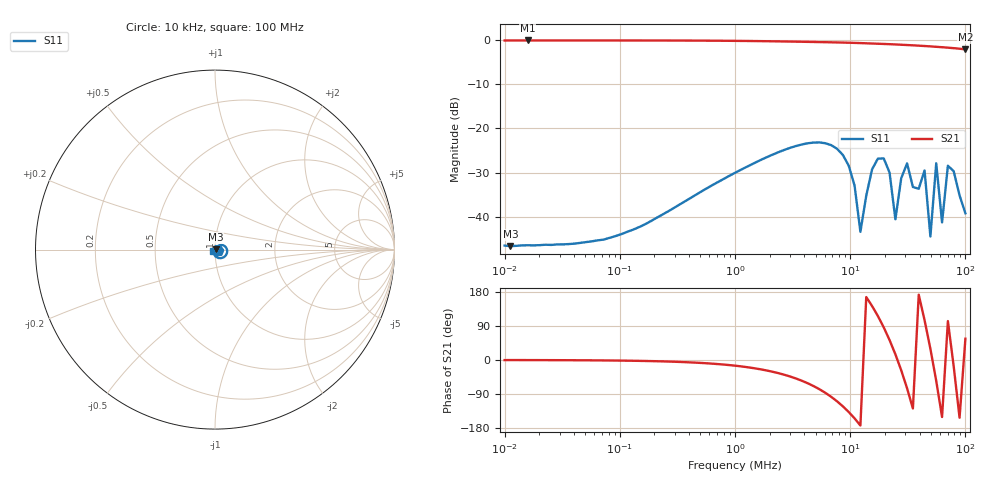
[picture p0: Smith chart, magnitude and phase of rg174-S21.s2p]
! ListType=Log
!!RG174 24.9f S21
# MHZ S RI R 50
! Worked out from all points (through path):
!   80 points, 10 kHz to 100 MHz, reference 50 ohm
!   highest |S21| = -0.09 dB at 15.94 kHz (marker M1); lowest = -2.1 dB at 100 MHz (marker M2)
!   lowest |S11| = -46.7 dB at 11.24 kHz (marker M3), VSWR 1.01, Z = 50.5 + j0.0596 ohm
!   |S11| at or under -10 dB: start of sweep to end of sweep
!   S12 and S22 are empty: the file has one direction only
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0.01  0.00469 0.000443  0.9886 -0.00335  0 0  0 0
0.0112365  0.0046 0.000591  0.9891 -0.0031  0 0  0 0
0.0159416  0.00471 0.000683  0.9892 -0.00432  0 0  0 0
0.0511518  0.00479 0.00192  0.9888 -0.0137  0 0  0 0
0.2328566  0.00646 0.0083  0.9858 -0.0622  0 0  0 0
1.060026  0.0228 0.0233  0.9409 -0.2672  0 0  0 0
4.825522  0.0677 -0.0138  0.3402 -0.8878  0 0  0 0
9.71274  0.00233 -0.0378  -0.685 -0.6324  0 0  0 0
12.26331  -0.00672 -0.000545  -0.9164 -0.1154  0 0  0 0
15.48365  0.0305 0.0157  -0.7242 0.5565  0 0  0 0
21.96707  0.00474 -0.0312  0.5452 0.7134  0 0  0 0
24.6834  -0.00934 -0.000571  0.8614 0.2302  0 0  0 0
31.16527  0.0386 -0.0109  0.233 -0.8464  0 0  0 0
39.34927  0.00594 0.0199  -0.8555 0.1163  0 0  0 0
44.215  0.0326 -0.00715  -0.2224 0.8261  0 0  0 0
49.6824  -0.000373 0.00596  0.737 0.4188  0 0  0 0
55.82586  0.0402 -0.00121  0.4791 -0.6879  0 0  0 0
62.729  -0.000702 0.00858  -0.7212 -0.4097  0 0  0 0
70.48574  0.0305 -0.0223  -0.1802 0.7992  0 0  0 0
79.20164  0.0263 0.0194  0.7723 -0.2412  0 0  0 0
88.9953  0.00271 0.0172  -0.7072 -0.3698  0 0  0 0
100  -0.0086 -0.00675  0.4353 0.6511  0 0  0 0
